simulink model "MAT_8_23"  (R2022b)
settings: Solver=ode45  StartTime=0.0  StopTime=10  RelTol=1e-3  EnableMultiTasking=on
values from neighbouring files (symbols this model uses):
  N = 5    [squarWave.m]    (also in gradient1.m = length(F))
undefined symbols (not defined in the file or in its folder): Kd, Ki, Kp

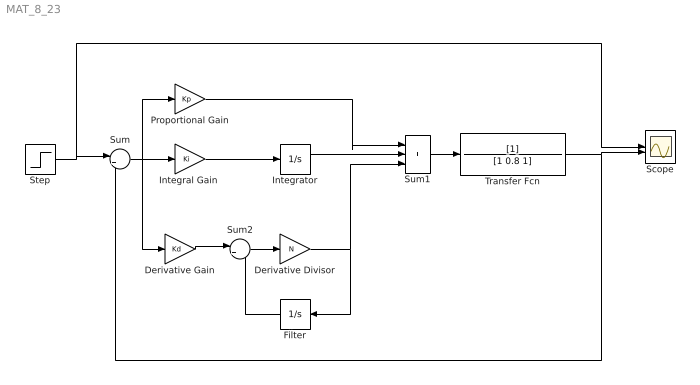
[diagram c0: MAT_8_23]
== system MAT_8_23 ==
  Derivative Divisor : Gain  Gain=N
  Derivative Gain : Gain  Gain=Kd
  Filter : Integrator
  "Integral Gain " : Gain  Gain=Ki
  Integrator : Integrator
  Proportional Gain : Gain  Gain=Kp
  Scope : Scope  NumInputPorts=2
  Step : Step  SampleTime=0
  Sum : Sum  Inputs=|+-
  Sum1 : Sum  Inputs=|+++
  Sum2 : Sum  Inputs=|+-
  Transfer Fcn : TransferFcn  Denominator=[1 0.8 1]
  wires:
  Step/1 -> Scope/1, Sum/1
  Sum/1 -> Proportional Gain/1, Derivative Gain/1, "Integral Gain "/1
  Transfer Fcn/1 -> Scope/2, Sum/2
  Sum1/1 -> Transfer Fcn/1
  "Integral Gain "/1 -> Integrator/1
  Integrator/1 -> Sum1/2
  Proportional Gain/1 -> Sum1/1
  Derivative Divisor/1 -> Sum1/3, Filter/1
  Filter/1 -> Sum2/2
  Sum2/1 -> Derivative Divisor/1
  Derivative Gain/1 -> Sum2/1
